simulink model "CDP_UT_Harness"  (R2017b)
settings: Solver=FixedStepDiscrete  StartTime=0.0  StopTime=10.0  FixedStep=0.01  RelTol=1e-3  EnableMultiTasking=on

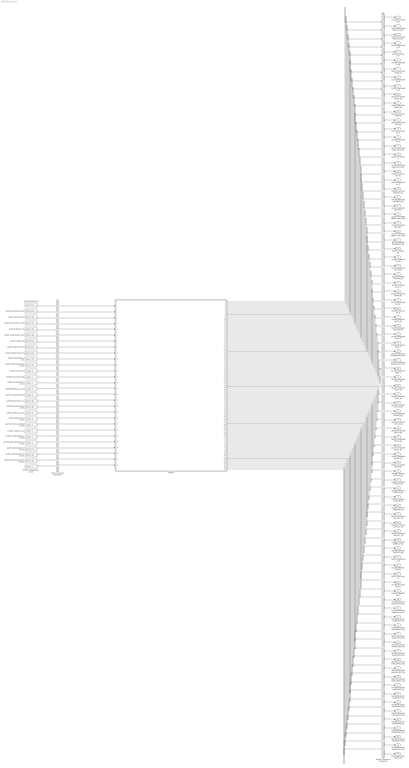
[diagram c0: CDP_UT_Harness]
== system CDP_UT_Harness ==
  CDP_UT : ModelReference  ModelNameDialog=CDP_UT  SimulationMode=Normal  ModelReferenceVersion='M110C20'
  GaISP_AFETempVld_numb : Constant  Value="zeros ( 8  , 1 )"  OutDataTypeStr=uint8  SampleTime=0.01
  GaISP_AFETemp_numb : Constant  Value="zeros ( 8  , 1 )"  OutDataTypeStr=fixdt('ufix16_Sp032_Bn273')  SampleTime=0.01
  GaISP_BusbarTempUpdCnt_numb : Constant  Value="zeros ( 48  , 1 )"  OutDataTypeStr=uint16  SampleTime=0.01
  GaISP_BusbarTempVld_numb : Constant  Value="zeros ( 48  , 1 )"  OutDataTypeStr=uint8  SampleTime=0.01
  GaISP_BusbarTemp_mV : Constant  Value="zeros ( 48  , 1 )"  OutDataTypeStr=uint16  SampleTime=0.01
  GaISP_CMUPCBTempVld_numb : Constant  Value="zeros ( 32  , 1 )"  OutDataTypeStr=uint8  SampleTime=0.01
  GaISP_CMUPCBTemp_mV : Constant  Value="zeros ( 32  , 1 )"  OutDataTypeStr=uint16  SampleTime=0.01
  GaISP_CellBalcOpLine_flg : Constant  Value="zeros ( 112  , 1 )"  OutDataTypeStr=boolean  SampleTime=0.01
  GaISP_CellBalcShrt_flg : Constant  Value="zeros ( 112  , 1 )"  OutDataTypeStr=boolean  SampleTime=0.01
  GaISP_CellBalc_flg : Constant  Value="zeros ( 112  , 1 )"  OutDataTypeStr=boolean  SampleTime=0.01
  GaISP_CellTempUpdCnt_numb : Constant  Value="zeros ( 48  , 1 )"  OutDataTypeStr=uint16  SampleTime=0.01
  GaISP_CellTempVld_numb : Constant  Value="zeros ( 48  , 1 )"  OutDataTypeStr=uint8  SampleTime=0.01
  GaISP_CellTemp_mV : Constant  Value="zeros ( 48  , 1 )"  OutDataTypeStr=uint16  SampleTime=0.01
  GaISP_CellVoltUpdCnt_numb : Constant  Value="zeros ( 112  , 1 )"  OutDataTypeStr=uint16  SampleTime=0.01
  GaISP_CellVoltVld_numb : Constant  Value="zeros ( 112  , 1 )"  OutDataTypeStr=uint8  SampleTime=0.01
  GaISP_CellVolt_mV : Constant  Value="zeros ( 112  , 1 )"  OutDataTypeStr=uint16  SampleTime=0.01
  GaISP_StackVoltVld_numb : Constant  Value="zeros ( 16  , 1 )"  OutDataTypeStr=uint8  SampleTime=0.01
  GaISP_StackVolt_mV : Constant  Value="zeros ( 16  , 1 )"  OutDataTypeStr=uint16  SampleTime=0.01
  GbCTC_ChrgHVMode_flg : Constant  Value="zeros ( 1  , 1 )"  OutDataTypeStr=boolean  SampleTime=0.01
  GbHDP_PackCrntVld_flg : Constant  Value="zeros ( 1  , 1 )"  OutDataTypeStr=boolean  SampleTime=0.01
  GcHDP_PackCrnt_A : Constant  Value="zeros ( 1  , 1 )"  OutDataTypeStr=single  SampleTime=0.01
  GcUDS_BusbarTempNumb_numb : Constant  Value="zeros ( 1  , 1 )"  OutDataTypeStr=uint8  SampleTime=0.01
  GcUDS_CellTempNumb_numb : Constant  Value="zeros ( 1  , 1 )"  OutDataTypeStr=uint8  SampleTime=0.01
  GcUDS_CellVoltNum_numb : Constant  Value="zeros ( 1  , 1 )"  OutDataTypeStr=uint8  SampleTime=0.01
  GeCTC_CtrCtlConnMode_enum : Constant  Value="zeros ( 1  , 1 )"  OutDataTypeStr=uint8  SampleTime=0.01
  GeISP_CmuReIninSts_enum : Constant  Value="zeros ( 1  , 1 )"  OutDataTypeStr=uint8  SampleTime=0.01
  GeMSM_BMUState_enum : Constant  Value="zeros ( 1  , 1 )"  OutDataTypeStr=uint8  SampleTime=0.01
  GeUDS_CapSel_enum : Constant  Value="zeros ( 1  , 1 )"  OutDataTypeStr=uint8  SampleTime=0.01
  Input Conversion Subsystem : Subsystem  Tag=__SLT_ICS__  Description=Signal spec. and routing
  Output Conversion Subsystem : Subsystem  Tag=__SLT_OCS__  Description=Signal spec. and routing
  GcCDP_SumCellVolt_V : Outport  OutDataTypeStr=single  PortDimensions=[1]
  GcCDP_MaxCellVoltNumb_numb : Outport  Port=2  OutDataTypeStr=uint8  PortDimensions=[1]
  GcCDP_MinCellVoltNumb_numb : Outport  Port=3  OutDataTypeStr=uint8  PortDimensions=[1]
  GcCDP_AvgCellVolt_mV : Outport  Port=4  OutDataTypeStr=uint16  PortDimensions=[1]
  GaCDP_CellVolt_mV : Outport  Port=5  OutDataTypeStr=uint16  PortDimensions=[112]
  GaCDP_CellVoltVld_flg : Outport  Port=6  OutDataTypeStr=boolean  PortDimensions=[112]
  GbCDP_SumCellVoltVld_flg : Outport  Port=7  OutDataTypeStr=boolean  PortDimensions=[1]
  GcCDP_MaxCellVolt_mV : Outport  Port=8  OutDataTypeStr=uint16  PortDimensions=[1]
  GcCDP_MinCellVolt_mV : Outport  Port=9  OutDataTypeStr=uint16  PortDimensions=[1]
  GbCDP_CellVoltSelfChck_flg : Outport  Port=10  OutDataTypeStr=boolean  PortDimensions=[1]
  GaCDP_StackVoltHighFlt_flg : Outport  Port=11  OutDataTypeStr=boolean  PortDimensions=[16]
  GaCDP_StackVoltLowFlt_flg : Outport  Port=12  OutDataTypeStr=boolean  PortDimensions=[16]
  GbCDP_AllCellTempVld_flg : Outport  Port=13  OutDataTypeStr=boolean  PortDimensions=[1]
  GcCDP_MaxCellTemp_C : Outport  Port=14  OutDataTypeStr=single  PortDimensions=[1]
  GcCDP_MinCellTemp_C : Outport  Port=15  OutDataTypeStr=single  PortDimensions=[1]
  GcCDP_MaxCellTempNumb_numb : Outport  Port=16  OutDataTypeStr=uint8  PortDimensions=[1]
  GaCDP_CellTemp_C : Outport  Port=17  OutDataTypeStr=single  PortDimensions=[48]
  GcCDP_MinCellTempNumb_numb : Outport  Port=18  OutDataTypeStr=uint8  PortDimensions=[1]
  GaCDP_CellTempVld_flg : Outport  Port=19  OutDataTypeStr=boolean  PortDimensions=[48]
  GcCDP_AvgCellTemp_C : Outport  Port=20  OutDataTypeStr=single  PortDimensions=[1]
  GbCDP_CellTempSelfChck_flg : Outport  Port=21  OutDataTypeStr=boolean  PortDimensions=[1]
  GaCDP_ModuleTempHighFlt_flg : Outport  Port=22  OutDataTypeStr=boolean  PortDimensions=[16]
  GcCDP_MaxCMUPCBTemp_C : Outport  Port=23  OutDataTypeStr=single  PortDimensions=[1]
  GcCDP_MaxCMUPCBTempNumb_numb : Outport  Port=24  OutDataTypeStr=uint8  PortDimensions=[1]
  GcCDP_MinCMUPCBTemp_C : Outport  Port=25  OutDataTypeStr=single  PortDimensions=[1]
  GcCDP_MinCMUPCBTempNumb_numb : Outport  Port=26  OutDataTypeStr=uint8  PortDimensions=[1]
  GbCDP_CMUPCBTempHighFlt_flg : Outport  Port=27  OutDataTypeStr=boolean  PortDimensions=[1]
  GaCDP_CellBalc_flg : Outport  Port=28  OutDataTypeStr=boolean  PortDimensions=[112]
  GaCDP_CellBalcShrt_flg : Outport  Port=29  OutDataTypeStr=boolean  PortDimensions=[112]
  GaCDP_CellBalcOpLine_flg : Outport  Port=30  OutDataTypeStr=boolean  PortDimensions=[112]
  GaCDP_CMUPCBTempVld_flg : Outport  Port=31  OutDataTypeStr=boolean  PortDimensions=[32]
  GaCDP_CMUPCBTemp_C : Outport  Port=32  OutDataTypeStr=single  PortDimensions=[32]
  GbCDP_SumModelVoltVld_flg : Outport  Port=33  OutDataTypeStr=boolean  PortDimensions=[1]
  GcCDP_SumModelVolt_V : Outport  Port=34  OutDataTypeStr=single  PortDimensions=[1]
  GaCDP_BusbarTemp_C : Outport  Port=35  OutDataTypeStr=single  PortDimensions=[48]
  GaCDP_BusbarTempVld_flg : Outport  Port=36  OutDataTypeStr=boolean  PortDimensions=[48]
  GbCDP_AllBusbarTempVld_flg : Outport  Port=37  OutDataTypeStr=boolean  PortDimensions=[1]
  GcCDP_MaxBusbarTemp_C : Outport  Port=38  OutDataTypeStr=single  PortDimensions=[1]
  GcCDP_MinBusbarTemp_C : Outport  Port=39  OutDataTypeStr=single  PortDimensions=[1]
  GcCDP_MaxBusbarTempNumb_numb : Outport  Port=40  OutDataTypeStr=uint8  PortDimensions=[1]
  GcCDP_MinBusbarTempNumb_numb : Outport  Port=41  OutDataTypeStr=uint8  PortDimensions=[1]
  GcCDP_AvgBusbarTemp_C : Outport  Port=42  OutDataTypeStr=single  PortDimensions=[1]
  GbCDP_CellVoltHiFltLv3_flg : Outport  Port=43  OutDataTypeStr=boolean  PortDimensions=[1]
  GbCDP_CellVoltHiFltLv2_flg : Outport  Port=44  OutDataTypeStr=boolean  PortDimensions=[1]
  GbCDP_CellVoltHiFltLv1_flg : Outport  Port=45  OutDataTypeStr=boolean  PortDimensions=[1]
  GbCDP_CellVoltLowFltLv3_flg : Outport  Port=46  OutDataTypeStr=boolean  PortDimensions=[1]
  GbCDP_CellVoltLowFltLv2_flg : Outport  Port=47  OutDataTypeStr=boolean  PortDimensions=[1]
  GbCDP_CellVoltLowFltLv1_flg : Outport  Port=48  OutDataTypeStr=boolean  PortDimensions=[1]
  GbCDP_CellVoltDiffFltLv3_flg : Outport  Port=49  OutDataTypeStr=boolean  PortDimensions=[1]
  GbCDP_CellVoltDiffFltLv2_flg : Outport  Port=50  OutDataTypeStr=boolean  PortDimensions=[1]
  GbCDP_CellVoltDiffFltLv1_flg : Outport  Port=51  OutDataTypeStr=boolean  PortDimensions=[1]
  GbCDP_CellVoltRngLowFlt_flg : Outport  Port=52  OutDataTypeStr=boolean  PortDimensions=[1]
  GbCDP_CellVoltRngHiFlt_flg : Outport  Port=53  OutDataTypeStr=boolean  PortDimensions=[1]
  GbCDP_CellTempHiFltLv3_flg : Outport  Port=54  OutDataTypeStr=boolean  PortDimensions=[1]
  GbCDP_CellTempHiFltLv2_flg : Outport  Port=55  OutDataTypeStr=boolean  PortDimensions=[1]
  GbCDP_CellTempHiFltLv1_flg : Outport  Port=56  OutDataTypeStr=boolean  PortDimensions=[1]
  GbCDP_CellTempRngHiFlt_flg : Outport  Port=57  OutDataTypeStr=boolean  PortDimensions=[1]
  GbCDP_CellTempRngLowFlt_flg : Outport  Port=58  OutDataTypeStr=boolean  PortDimensions=[1]
  GbCDP_CellTempLowFltLv3_flg : Outport  Port=59  OutDataTypeStr=boolean  PortDimensions=[1]
  GbCDP_CellTempLowFltLv2_flg : Outport  Port=60  OutDataTypeStr=boolean  PortDimensions=[1]
  GbCDP_CellTempLowFltLv1_flg : Outport  Port=61  OutDataTypeStr=boolean  PortDimensions=[1]
  GbCDP_CellTempDiffFltLv2_flg : Outport  Port=62  OutDataTypeStr=boolean  PortDimensions=[1]
  GbCDP_CellTempDiffFltLv1_flg : Outport  Port=63  OutDataTypeStr=boolean  PortDimensions=[1]
  GaCDP_ModuleVolt_mV : Outport  Port=64  OutDataTypeStr=uint16  PortDimensions=[16]
  GaCDP_AFETempVld_flg : Outport  Port=65  OutDataTypeStr=boolean  PortDimensions=[8]
  GaCDP_AFETemp_C : Outport  Port=66  OutDataTypeStr=single  PortDimensions=[8]
  GcCDP_MaxAFETemp_C : Outport  Port=67  OutDataTypeStr=single  PortDimensions=[1]
  GcCDP_MinAFETemp_C : Outport  Port=68  OutDataTypeStr=single  PortDimensions=[1]
  GcCDP_MaxAFETempNumb_numb : Outport  Port=69  OutDataTypeStr=uint8  PortDimensions=[1]
  GcCDP_MinAFETempNumb_numb : Outport  Port=70  OutDataTypeStr=uint8  PortDimensions=[1]
  GbCDP_BusbarTempHiFltLv3_flg : Outport  Port=71  OutDataTypeStr=boolean  PortDimensions=[1]
  GbCDP_BusbarTempLowFltLv3_flg : Outport  Port=72  OutDataTypeStr=boolean  PortDimensions=[1]
  GbCDP_ChrgCellTempHiFltLv3_flg : Outport  Port=73  OutDataTypeStr=boolean  PortDimensions=[1]
  GbCDP_ChrgCellTempHiFltLv2_flg : Outport  Port=74  OutDataTypeStr=boolean  PortDimensions=[1]
  GbCDP_ChrgCellTempHiFltLv1_flg : Outport  Port=75  OutDataTypeStr=boolean  PortDimensions=[1]
  GbCDP_ChrgCellTempLowFltLv3_flg : Outport  Port=76  OutDataTypeStr=boolean  PortDimensions=[1]
  GbCDP_ChrgCellTempLowFltLv2_flg : Outport  Port=77  OutDataTypeStr=boolean  PortDimensions=[1]
  GbCDP_ChrgCellTempLowFltLv1_flg : Outport  Port=78  OutDataTypeStr=boolean  PortDimensions=[1]
  GbCDP_BusbarTempHiFltLv2_flg : Outport  Port=79  OutDataTypeStr=boolean  PortDimensions=[1]
  GbCDP_BusbarTempHiFltLv1_flg : Outport  Port=80  OutDataTypeStr=boolean  PortDimensions=[1]
  GbCDP_BusbarTempLowFltLv2_flg : Outport  Port=81  OutDataTypeStr=boolean  PortDimensions=[1]
  GbCDP_BusbarTempLowFltLv1_flg : Outport  Port=82  OutDataTypeStr=boolean  PortDimensions=[1]
  GbCDP_BusbarTempRngHiFlt_flg : Outport  Port=83  OutDataTypeStr=boolean  PortDimensions=[1]
  GbCDP_BusbarTempRngLowFlt_flg : Outport  Port=84  OutDataTypeStr=boolean  PortDimensions=[1]
  GbCDP_BusbarTempDiffFltLv2_flg : Outport  Port=85  OutDataTypeStr=boolean  PortDimensions=[1]
  GbCDP_BusbarTempDiffFltLv1_flg : Outport  Port=86  OutDataTypeStr=boolean  PortDimensions=[1]
  GbCDP_AFETempHighFlt_flg : Outport  Port=87  OutDataTypeStr=boolean  PortDimensions=[1]
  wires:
  GaISP_CellVolt_mV/1 -> Input Conversion Subsystem/1(Inport_1)
  GaISP_CellVoltVld_numb/1 -> Input Conversion Subsystem/2(Inport_2)
  GaISP_StackVolt_mV/1 -> Input Conversion Subsystem/3(Inport_3)
  GaISP_StackVoltVld_numb/1 -> Input Conversion Subsystem/4(Inport_4)
  GaISP_CellTemp_mV/1 -> Input Conversion Subsystem/5(Inport_5)
  GaISP_CellTempVld_numb/1 -> Input Conversion Subsystem/6(Inport_6)
  GaISP_CellBalc_flg/1 -> Input Conversion Subsystem/7(Inport_7)
  GaISP_CellBalcShrt_flg/1 -> Input Conversion Subsystem/8(Inport_8)
  GaISP_CellBalcOpLine_flg/1 -> Input Conversion Subsystem/9(Inport_9)
  GaISP_CMUPCBTemp_mV/1 -> Input Conversion Subsystem/10(Inport_10)
  GaISP_CMUPCBTempVld_numb/1 -> Input Conversion Subsystem/11(Inport_11)
  GcHDP_PackCrnt_A/1 -> Input Conversion Subsystem/12(Inport_12)
  GbHDP_PackCrntVld_flg/1 -> Input Conversion Subsystem/13(Inport_13)
  GeISP_CmuReIninSts_enum/1 -> Input Conversion Subsystem/14(Inport_14)
  GeMSM_BMUState_enum/1 -> Input Conversion Subsystem/15(Inport_15)
  GbCTC_ChrgHVMode_flg/1 -> Input Conversion Subsystem/16(Inport_16)
  GaISP_BusbarTemp_mV/1 -> Input Conversion Subsystem/17(Inport_17)
  GaISP_BusbarTempVld_numb/1 -> Input Conversion Subsystem/18(Inport_18)
  GaISP_AFETemp_numb/1 -> Input Conversion Subsystem/19(Inport_19)
  GaISP_AFETempVld_numb/1 -> Input Conversion Subsystem/20(Inport_20)
  GeCTC_CtrCtlConnMode_enum/1 -> Input Conversion Subsystem/21(Inport_21)
  GeUDS_CapSel_enum/1 -> Input Conversion Subsystem/22(Inport_22)
  GcUDS_CellTempNumb_numb/1 -> Input Conversion Subsystem/23(Inport_23)
  GcUDS_BusbarTempNumb_numb/1 -> Input Conversion Subsystem/24(Inport_24)
  GaISP_CellVoltUpdCnt_numb/1 -> Input Conversion Subsystem/25(Inport_25)
  GaISP_CellTempUpdCnt_numb/1 -> Input Conversion Subsystem/26(Inport_26)
  GaISP_BusbarTempUpdCnt_numb/1 -> Input Conversion Subsystem/27(Inport_27)
  GcUDS_CellVoltNum_numb/1 -> Input Conversion Subsystem/28(Inport_28)
  Output Conversion Subsystem/1(Outport_1) -> GcCDP_SumCellVolt_V/1
  Output Conversion Subsystem/2(Outport_2) -> GcCDP_MaxCellVoltNumb_numb/1
  Output Conversion Subsystem/3(Outport_3) -> GcCDP_MinCellVoltNumb_numb/1
  Output Conversion Subsystem/4(Outport_4) -> GcCDP_AvgCellVolt_mV/1
  Output Conversion Subsystem/5(Outport_5) -> GaCDP_CellVolt_mV/1
  Output Conversion Subsystem/6(Outport_6) -> GaCDP_CellVoltVld_flg/1
  Output Conversion Subsystem/7(Outport_7) -> GbCDP_SumCellVoltVld_flg/1
  Output Conversion Subsystem/8(Outport_8) -> GcCDP_MaxCellVolt_mV/1
  Output Conversion Subsystem/9(Outport_9) -> GcCDP_MinCellVolt_mV/1
  Output Conversion Subsystem/10(Outport_10) -> GbCDP_CellVoltSelfChck_flg/1
  Output Conversion Subsystem/11(Outport_11) -> GaCDP_StackVoltHighFlt_flg/1
  Output Conversion Subsystem/12(Outport_12) -> GaCDP_StackVoltLowFlt_flg/1
  Output Conversion Subsystem/13(Outport_13) -> GbCDP_AllCellTempVld_flg/1
  Output Conversion Subsystem/14(Outport_14) -> GcCDP_MaxCellTemp_C/1
  Output Conversion Subsystem/15(Outport_15) -> GcCDP_MinCellTemp_C/1
  Output Conversion Subsystem/16(Outport_16) -> GcCDP_MaxCellTempNumb_numb/1
  Output Conversion Subsystem/17(Outport_17) -> GaCDP_CellTemp_C/1
  Output Conversion Subsystem/18(Outport_18) -> GcCDP_MinCellTempNumb_numb/1
  Output Conversion Subsystem/19(Outport_19) -> GaCDP_CellTempVld_flg/1
  Output Conversion Subsystem/20(Outport_20) -> GcCDP_AvgCellTemp_C/1
  Output Conversion Subsystem/21(Outport_21) -> GbCDP_CellTempSelfChck_flg/1
  Output Conversion Subsystem/22(Outport_22) -> GaCDP_ModuleTempHighFlt_flg/1
  Output Conversion Subsystem/23(Outport_23) -> GcCDP_MaxCMUPCBTemp_C/1
  Output Conversion Subsystem/24(Outport_24) -> GcCDP_MaxCMUPCBTempNumb_numb/1
  Output Conversion Subsystem/25(Outport_25) -> GcCDP_MinCMUPCBTemp_C/1
  Output Conversion Subsystem/26(Outport_26) -> GcCDP_MinCMUPCBTempNumb_numb/1
  Output Conversion Subsystem/27(Outport_27) -> GbCDP_CMUPCBTempHighFlt_flg/1
  Output Conversion Subsystem/28(Outport_28) -> GaCDP_CellBalc_flg/1
  Output Conversion Subsystem/29(Outport_29) -> GaCDP_CellBalcShrt_flg/1
  Output Conversion Subsystem/30(Outport_30) -> GaCDP_CellBalcOpLine_flg/1
  Output Conversion Subsystem/31(Outport_31) -> GaCDP_CMUPCBTempVld_flg/1
  Output Conversion Subsystem/32(Outport_32) -> GaCDP_CMUPCBTemp_C/1
  Output Conversion Subsystem/33(Outport_33) -> GbCDP_SumModelVoltVld_flg/1
  Output Conversion Subsystem/34(Outport_34) -> GcCDP_SumModelVolt_V/1
  Output Conversion Subsystem/35(Outport_35) -> GaCDP_BusbarTemp_C/1
  Output Conversion Subsystem/36(Outport_36) -> GaCDP_BusbarTempVld_flg/1
  Output Conversion Subsystem/37(Outport_37) -> GbCDP_AllBusbarTempVld_flg/1
  Output Conversion Subsystem/38(Outport_38) -> GcCDP_MaxBusbarTemp_C/1
  Output Conversion Subsystem/39(Outport_39) -> GcCDP_MinBusbarTemp_C/1
  Output Conversion Subsystem/40(Outport_40) -> GcCDP_MaxBusbarTempNumb_numb/1
  Output Conversion Subsystem/41(Outport_41) -> GcCDP_MinBusbarTempNumb_numb/1
  Output Conversion Subsystem/42(Outport_42) -> GcCDP_AvgBusbarTemp_C/1
  Output Conversion Subsystem/43(Outport_43) -> GbCDP_CellVoltHiFltLv3_flg/1
  Output Conversion Subsystem/44(Outport_44) -> GbCDP_CellVoltHiFltLv2_flg/1
  Output Conversion Subsystem/45(Outport_45) -> GbCDP_CellVoltHiFltLv1_flg/1
  Output Conversion Subsystem/46(Outport_46) -> GbCDP_CellVoltLowFltLv3_flg/1
  Output Conversion Subsystem/47(Outport_47) -> GbCDP_CellVoltLowFltLv2_flg/1
  Output Conversion Subsystem/48(Outport_48) -> GbCDP_CellVoltLowFltLv1_flg/1
  Output Conversion Subsystem/49(Outport_49) -> GbCDP_CellVoltDiffFltLv3_flg/1
  Output Conversion Subsystem/50(Outport_50) -> GbCDP_CellVoltDiffFltLv2_flg/1
  Output Conversion Subsystem/51(Outport_51) -> GbCDP_CellVoltDiffFltLv1_flg/1
  Output Conversion Subsystem/52(Outport_52) -> GbCDP_CellVoltRngLowFlt_flg/1
  Output Conversion Subsystem/53(Outport_53) -> GbCDP_CellVoltRngHiFlt_flg/1
  Output Conversion Subsystem/54(Outport_54) -> GbCDP_CellTempHiFltLv3_flg/1
  Output Conversion Subsystem/55(Outport_55) -> GbCDP_CellTempHiFltLv2_flg/1
  Output Conversion Subsystem/56(Outport_56) -> GbCDP_CellTempHiFltLv1_flg/1
  Output Conversion Subsystem/57(Outport_57) -> GbCDP_CellTempRngHiFlt_flg/1
  Output Conversion Subsystem/58(Outport_58) -> GbCDP_CellTempRngLowFlt_flg/1
  Output Conversion Subsystem/59(Outport_59) -> GbCDP_CellTempLowFltLv3_flg/1
  Output Conversion Subsystem/60(Outport_60) -> GbCDP_CellTempLowFltLv2_flg/1
  Output Conversion Subsystem/61(Outport_61) -> GbCDP_CellTempLowFltLv1_flg/1
  Output Conversion Subsystem/62(Outport_62) -> GbCDP_CellTempDiffFltLv2_flg/1
  Output Conversion Subsystem/63(Outport_63) -> GbCDP_CellTempDiffFltLv1_flg/1
  Output Conversion Subsystem/64(Outport_64) -> GaCDP_ModuleVolt_mV/1
  Output Conversion Subsystem/65(Outport_65) -> GaCDP_AFETempVld_flg/1
  Output Conversion Subsystem/66(Outport_66) -> GaCDP_AFETemp_C/1
  Output Conversion Subsystem/67(Outport_67) -> GcCDP_MaxAFETemp_C/1
  Output Conversion Subsystem/68(Outport_68) -> GcCDP_MinAFETemp_C/1
  Output Conversion Subsystem/69(Outport_69) -> GcCDP_MaxAFETempNumb_numb/1
  Output Conversion Subsystem/70(Outport_70) -> GcCDP_MinAFETempNumb_numb/1
  Output Conversion Subsystem/71(Outport_71) -> GbCDP_BusbarTempHiFltLv3_flg/1
  Output Conversion Subsystem/72(Outport_72) -> GbCDP_BusbarTempLowFltLv3_flg/1
  Output Conversion Subsystem/73(Outport_73) -> GbCDP_ChrgCellTempHiFltLv3_flg/1
  Output Conversion Subsystem/74(Outport_74) -> GbCDP_ChrgCellTempHiFltLv2_flg/1
  Output Conversion Subsystem/75(Outport_75) -> GbCDP_ChrgCellTempHiFltLv1_flg/1
  Output Conversion Subsystem/76(Outport_76) -> GbCDP_ChrgCellTempLowFltLv3_flg/1
  Output Conversion Subsystem/77(Outport_77) -> GbCDP_ChrgCellTempLowFltLv2_flg/1
  Output Conversion Subsystem/78(Outport_78) -> GbCDP_ChrgCellTempLowFltLv1_flg/1
  Output Conversion Subsystem/79(Outport_79) -> GbCDP_BusbarTempHiFltLv2_flg/1
  Output Conversion Subsystem/80(Outport_80) -> GbCDP_BusbarTempHiFltLv1_flg/1
  Output Conversion Subsystem/81(Outport_81) -> GbCDP_BusbarTempLowFltLv2_flg/1
  Output Conversion Subsystem/82(Outport_82) -> GbCDP_BusbarTempLowFltLv1_flg/1
  Output Conversion Subsystem/83(Outport_83) -> GbCDP_BusbarTempRngHiFlt_flg/1
  Output Conversion Subsystem/84(Outport_84) -> GbCDP_BusbarTempRngLowFlt_flg/1
  Output Conversion Subsystem/85(Outport_85) -> GbCDP_BusbarTempDiffFltLv2_flg/1
  Output Conversion Subsystem/86(Outport_86) -> GbCDP_BusbarTempDiffFltLv1_flg/1
  Output Conversion Subsystem/87(Outport_87) -> GbCDP_AFETempHighFlt_flg/1
  Input Conversion Subsystem/1(Outport_1) -> CDP_UT/1
  Input Conversion Subsystem/2(Outport_2) -> CDP_UT/2
  Input Conversion Subsystem/3(Outport_3) -> CDP_UT/3
  Input Conversion Subsystem/4(Outport_4) -> CDP_UT/4
  Input Conversion Subsystem/5(Outport_5) -> CDP_UT/5
  Input Conversion Subsystem/6(Outport_6) -> CDP_UT/6
  Input Conversion Subsystem/7(Outport_7) -> CDP_UT/7
  Input Conversion Subsystem/8(Outport_8) -> CDP_UT/8
  Input Conversion Subsystem/9(Outport_9) -> CDP_UT/9
  Input Conversion Subsystem/10(Outport_10) -> CDP_UT/10
  Input Conversion Subsystem/11(Outport_11) -> CDP_UT/11
  Input Conversion Subsystem/12(Outport_12) -> CDP_UT/12
  Input Conversion Subsystem/13(Outport_13) -> CDP_UT/13
  Input Conversion Subsystem/14(Outport_14) -> CDP_UT/14
  Input Conversion Subsystem/15(Outport_15) -> CDP_UT/15
  Input Conversion Subsystem/16(Outport_16) -> CDP_UT/16
  Input Conversion Subsystem/17(Outport_17) -> CDP_UT/17
  Input Conversion Subsystem/18(Outport_18) -> CDP_UT/18
  Input Conversion Subsystem/19(Outport_19) -> CDP_UT/19
  Input Conversion Subsystem/20(Outport_20) -> CDP_UT/20
  Input Conversion Subsystem/21(Outport_21) -> CDP_UT/21
  Input Conversion Subsystem/22(Outport_22) -> CDP_UT/22
  Input Conversion Subsystem/23(Outport_23) -> CDP_UT/23
  Input Conversion Subsystem/24(Outport_24) -> CDP_UT/24
  Input Conversion Subsystem/25(Outport_25) -> CDP_UT/25
  Input Conversion Subsystem/26(Outport_26) -> CDP_UT/26
  Input Conversion Subsystem/27(Outport_27) -> CDP_UT/27
  Input Conversion Subsystem/28(Outport_28) -> CDP_UT/28
  CDP_UT/1 -> Output Conversion Subsystem/1(Inport_1)
  CDP_UT/2 -> Output Conversion Subsystem/2(Inport_2)
  CDP_UT/3 -> Output Conversion Subsystem/3(Inport_3)
  CDP_UT/4 -> Output Conversion Subsystem/4(Inport_4)
  CDP_UT/5 -> Output Conversion Subsystem/5(Inport_5)
  CDP_UT/6 -> Output Conversion Subsystem/6(Inport_6)
  CDP_UT/7 -> Output Conversion Subsystem/7(Inport_7)
  CDP_UT/8 -> Output Conversion Subsystem/8(Inport_8)
  CDP_UT/9 -> Output Conversion Subsystem/9(Inport_9)
  CDP_UT/10 -> Output Conversion Subsystem/10(Inport_10)
  CDP_UT/11 -> Output Conversion Subsystem/11(Inport_11)
  CDP_UT/12 -> Output Conversion Subsystem/12(Inport_12)
  CDP_UT/13 -> Output Conversion Subsystem/13(Inport_13)
  CDP_UT/14 -> Output Conversion Subsystem/14(Inport_14)
  CDP_UT/15 -> Output Conversion Subsystem/15(Inport_15)
  CDP_UT/16 -> Output Conversion Subsystem/16(Inport_16)
  CDP_UT/17 -> Output Conversion Subsystem/17(Inport_17)
  CDP_UT/18 -> Output Conversion Subsystem/18(Inport_18)
  CDP_UT/19 -> Output Conversion Subsystem/19(Inport_19)
  CDP_UT/20 -> Output Conversion Subsystem/20(Inport_20)
  CDP_UT/21 -> Output Conversion Subsystem/21(Inport_21)
  CDP_UT/22 -> Output Conversion Subsystem/22(Inport_22)
  CDP_UT/23 -> Output Conversion Subsystem/23(Inport_23)
  CDP_UT/24 -> Output Conversion Subsystem/24(Inport_24)
  CDP_UT/25 -> Output Conversion Subsystem/25(Inport_25)
  CDP_UT/26 -> Output Conversion Subsystem/26(Inport_26)
  CDP_UT/27 -> Output Conversion Subsystem/27(Inport_27)
  CDP_UT/28 -> Output Conversion Subsystem/28(Inport_28)
  CDP_UT/29 -> Output Conversion Subsystem/29(Inport_29)
  CDP_UT/30 -> Output Conversion Subsystem/30(Inport_30)
  CDP_UT/31 -> Output Conversion Subsystem/31(Inport_31)
  CDP_UT/32 -> Output Conversion Subsystem/32(Inport_32)
  CDP_UT/33 -> Output Conversion Subsystem/33(Inport_33)
  CDP_UT/34 -> Output Conversion Subsystem/34(Inport_34)
  CDP_UT/35 -> Output Conversion Subsystem/35(Inport_35)
  CDP_UT/36 -> Output Conversion Subsystem/36(Inport_36)
  CDP_UT/37 -> Output Conversion Subsystem/37(Inport_37)
  CDP_UT/38 -> Output Conversion Subsystem/38(Inport_38)
  CDP_UT/39 -> Output Conversion Subsystem/39(Inport_39)
  CDP_UT/40 -> Output Conversion Subsystem/40(Inport_40)
  CDP_UT/41 -> Output Conversion Subsystem/41(Inport_41)
  CDP_UT/42 -> Output Conversion Subsystem/42(Inport_42)
  CDP_UT/43 -> Output Conversion Subsystem/43(Inport_43)
  CDP_UT/44 -> Output Conversion Subsystem/44(Inport_44)
  CDP_UT/45 -> Output Conversion Subsystem/45(Inport_45)
  CDP_UT/46 -> Output Conversion Subsystem/46(Inport_46)
  CDP_UT/47 -> Output Conversion Subsystem/47(Inport_47)
  CDP_UT/48 -> Output Conversion Subsystem/48(Inport_48)
  CDP_UT/49 -> Output Conversion Subsystem/49(Inport_49)
  CDP_UT/50 -> Output Conversion Subsystem/50(Inport_50)
  CDP_UT/51 -> Output Conversion Subsystem/51(Inport_51)
  CDP_UT/52 -> Output Conversion Subsystem/52(Inport_52)
  CDP_UT/53 -> Output Conversion Subsystem/53(Inport_53)
  CDP_UT/54 -> Output Conversion Subsystem/54(Inport_54)
  CDP_UT/55 -> Output Conversion Subsystem/55(Inport_55)
  CDP_UT/56 -> Output Conversion Subsystem/56(Inport_56)
  CDP_UT/57 -> Output Conversion Subsystem/57(Inport_57)
  CDP_UT/58 -> Output Conversion Subsystem/58(Inport_58)
  CDP_UT/59 -> Output Conversion Subsystem/59(Inport_59)
  CDP_UT/60 -> Output Conversion Subsystem/60(Inport_60)
  CDP_UT/61 -> Output Conversion Subsystem/61(Inport_61)
  CDP_UT/62 -> Output Conversion Subsystem/62(Inport_62)
  CDP_UT/63 -> Output Conversion Subsystem/63(Inport_63)
  CDP_UT/64 -> Output Conversion Subsystem/64(Inport_64)
  CDP_UT/65 -> Output Conversion Subsystem/65(Inport_65)
  CDP_UT/66 -> Output Conversion Subsystem/66(Inport_66)
  CDP_UT/67 -> Output Conversion Subsystem/67(Inport_67)
  CDP_UT/68 -> Output Conversion Subsystem/68(Inport_68)
  CDP_UT/69 -> Output Conversion Subsystem/69(Inport_69)
  CDP_UT/70 -> Output Conversion Subsystem/70(Inport_70)
  CDP_UT/71 -> Output Conversion Subsystem/71(Inport_71)
  CDP_UT/72 -> Output Conversion Subsystem/72(Inport_72)
  CDP_UT/73 -> Output Conversion Subsystem/73(Inport_73)
  CDP_UT/74 -> Output Conversion Subsystem/74(Inport_74)
  CDP_UT/75 -> Output Conversion Subsystem/75(Inport_75)
  CDP_UT/76 -> Output Conversion Subsystem/76(Inport_76)
  CDP_UT/77 -> Output Conversion Subsystem/77(Inport_77)
  CDP_UT/78 -> Output Conversion Subsystem/78(Inport_78)
  CDP_UT/79 -> Output Conversion Subsystem/79(Inport_79)
  CDP_UT/80 -> Output Conversion Subsystem/80(Inport_80)
  CDP_UT/81 -> Output Conversion Subsystem/81(Inport_81)
  CDP_UT/82 -> Output Conversion Subsystem/82(Inport_82)
  CDP_UT/83 -> Output Conversion Subsystem/83(Inport_83)
  CDP_UT/84 -> Output Conversion Subsystem/84(Inport_84)
  CDP_UT/85 -> Output Conversion Subsystem/85(Inport_85)
  CDP_UT/86 -> Output Conversion Subsystem/86(Inport_86)
  CDP_UT/87 -> Output Conversion Subsystem/87(Inport_87)

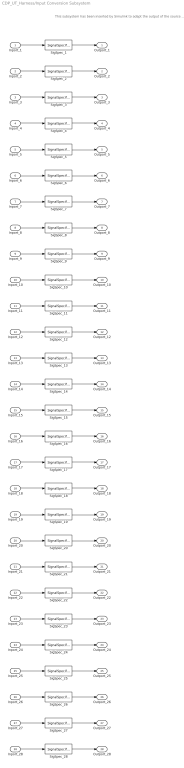
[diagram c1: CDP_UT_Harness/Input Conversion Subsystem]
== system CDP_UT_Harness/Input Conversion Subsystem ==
  note: This subsystem has been inserted by Simulink to adapt the output of the source blocks to the interface required by the harnessed component. Modifying the contents of this subsystem may result in compilation and simulation failure.
  Inport_1 : Inport
  Inport_2 : Inport  Port=2
  Inport_3 : Inport  Port=3
  Inport_4 : Inport  Port=4
  Inport_5 : Inport  Port=5
  Inport_6 : Inport  Port=6
  Inport_7 : Inport  Port=7
  Inport_8 : Inport  Port=8
  Inport_9 : Inport  Port=9
  Inport_10 : Inport  Port=10
  Inport_11 : Inport  Port=11
  Inport_12 : Inport  Port=12
  Inport_13 : Inport  Port=13
  Inport_14 : Inport  Port=14
  Inport_15 : Inport  Port=15
  Inport_16 : Inport  Port=16
  Inport_17 : Inport  Port=17
  Inport_18 : Inport  Port=18
  Inport_19 : Inport  Port=19
  Inport_20 : Inport  Port=20
  Inport_21 : Inport  Port=21
  Inport_22 : Inport  Port=22
  Inport_23 : Inport  Port=23
  Inport_24 : Inport  Port=24
  Inport_25 : Inport  Port=25
  Inport_26 : Inport  Port=26
  Inport_27 : Inport  Port=27
  Inport_28 : Inport  Port=28
  SigSpec_1 : SignalSpecification  OutDataTypeStr=uint16  Unit=mV  Dimensions=[112]  SampleTime=0.01
  SigSpec_10 : SignalSpecification  OutDataTypeStr=uint16  Unit=mV  Dimensions=[32]  SampleTime=0.01
  SigSpec_11 : SignalSpecification  OutDataTypeStr=uint8  Unit=numb  Dimensions=[32]  SampleTime=0.01
  SigSpec_12 : SignalSpecification  OutDataTypeStr=single  Unit=A  Dimensions=[1]  SampleTime=0.01
  SigSpec_13 : SignalSpecification  OutDataTypeStr=boolean  Unit=flag  Dimensions=[1]  SampleTime=0.01
  SigSpec_{14..15,21..22} (4 alike) : SignalSpecification  OutDataTypeStr=uint8  Unit=enum  Dimensions=[1]  SampleTime=0.01
  SigSpec_16 : SignalSpecification  OutDataTypeStr=boolean  Unit=flag  Dimensions=[1]  SampleTime=0.01
  SigSpec_17 : SignalSpecification  OutDataTypeStr=uint16  Unit=mV  Dimensions=[48]  SampleTime=0.01
  SigSpec_18 : SignalSpecification  OutDataTypeStr=uint8  Unit=numb  Dimensions=[48]  SampleTime=0.01
  SigSpec_19 : SignalSpecification  OutDataTypeStr=fixdt('ufix16_Sp032_Bn273')  Unit=numb  Dimensions=[8]  SampleTime=0.01
  SigSpec_2 : SignalSpecification  OutDataTypeStr=uint8  Unit=numb  Dimensions=[112]  SampleTime=0.01
  SigSpec_20 : SignalSpecification  OutDataTypeStr=uint8  Unit=numb  Dimensions=[8]  SampleTime=0.01
  SigSpec_23 : SignalSpecification  OutDataTypeStr=uint8  Unit=numb  Dimensions=[1]  SampleTime=0.01
  SigSpec_24 : SignalSpecification  OutDataTypeStr=uint8  Unit=numb  Dimensions=[1]  SampleTime=0.01
  SigSpec_25 : SignalSpecification  OutDataTypeStr=uint16  Unit=numb  Dimensions=[112]  SampleTime=0.01
  SigSpec_26 : SignalSpecification  OutDataTypeStr=uint16  Unit=numb  Dimensions=[48]  SampleTime=0.01
  SigSpec_27 : SignalSpecification  OutDataTypeStr=uint16  Unit=numb  Dimensions=[48]  SampleTime=0.01
  SigSpec_28 : SignalSpecification  OutDataTypeStr=uint8  Unit=numb  Dimensions=[1]  SampleTime=0.01
  SigSpec_3 : SignalSpecification  OutDataTypeStr=uint16  Unit=mV  Dimensions=[16]  SampleTime=0.01
  SigSpec_4 : SignalSpecification  OutDataTypeStr=uint8  Unit=numb  Dimensions=[16]  SampleTime=0.01
  SigSpec_5 : SignalSpecification  OutDataTypeStr=uint16  Unit=mV  Dimensions=[48]  SampleTime=0.01
  SigSpec_6 : SignalSpecification  OutDataTypeStr=uint8  Unit=numb  Dimensions=[48]  SampleTime=0.01
  SigSpec_7 : SignalSpecification  OutDataTypeStr=boolean  Unit=flag  Dimensions=[112]  SampleTime=0.01
  SigSpec_8 : SignalSpecification  OutDataTypeStr=boolean  Unit=flag  Dimensions=[112]  SampleTime=0.01
  SigSpec_9 : SignalSpecification  OutDataTypeStr=boolean  Unit=flag  Dimensions=[112]  SampleTime=0.01
  Outport_1 : Outport
  Outport_2 : Outport  Port=2
  Outport_3 : Outport  Port=3
  Outport_4 : Outport  Port=4
  Outport_5 : Outport  Port=5
  Outport_6 : Outport  Port=6
  Outport_7 : Outport  Port=7
  Outport_8 : Outport  Port=8
  Outport_9 : Outport  Port=9
  Outport_10 : Outport  Port=10
  Outport_11 : Outport  Port=11
  Outport_12 : Outport  Port=12
  Outport_13 : Outport  Port=13
  Outport_14 : Outport  Port=14
  Outport_15 : Outport  Port=15
  Outport_16 : Outport  Port=16
  Outport_17 : Outport  Port=17
  Outport_18 : Outport  Port=18
  Outport_19 : Outport  Port=19
  Outport_20 : Outport  Port=20
  Outport_21 : Outport  Port=21
  Outport_22 : Outport  Port=22
  Outport_23 : Outport  Port=23
  Outport_24 : Outport  Port=24
  Outport_25 : Outport  Port=25
  Outport_26 : Outport  Port=26
  Outport_27 : Outport  Port=27
  Outport_28 : Outport  Port=28
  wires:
  SigSpec_1/1 -> Outport_1/1
  Inport_1/1 -> SigSpec_1/1
  SigSpec_2/1 -> Outport_2/1
  Inport_2/1 -> SigSpec_2/1
  SigSpec_3/1 -> Outport_3/1
  Inport_3/1 -> SigSpec_3/1
  SigSpec_4/1 -> Outport_4/1
  Inport_4/1 -> SigSpec_4/1
  SigSpec_5/1 -> Outport_5/1
  Inport_5/1 -> SigSpec_5/1
  SigSpec_6/1 -> Outport_6/1
  Inport_6/1 -> SigSpec_6/1
  SigSpec_7/1 -> Outport_7/1
  Inport_7/1 -> SigSpec_7/1
  SigSpec_8/1 -> Outport_8/1
  Inport_8/1 -> SigSpec_8/1
  SigSpec_9/1 -> Outport_9/1
  Inport_9/1 -> SigSpec_9/1
  SigSpec_10/1 -> Outport_10/1
  Inport_10/1 -> SigSpec_10/1
  SigSpec_11/1 -> Outport_11/1
  Inport_11/1 -> SigSpec_11/1
  SigSpec_12/1 -> Outport_12/1
  Inport_12/1 -> SigSpec_12/1
  SigSpec_13/1 -> Outport_13/1
  Inport_13/1 -> SigSpec_13/1
  SigSpec_14/1 -> Outport_14/1
  Inport_14/1 -> SigSpec_14/1
  SigSpec_15/1 -> Outport_15/1
  Inport_15/1 -> SigSpec_15/1
  SigSpec_16/1 -> Outport_16/1
  Inport_16/1 -> SigSpec_16/1
  SigSpec_17/1 -> Outport_17/1
  Inport_17/1 -> SigSpec_17/1
  SigSpec_18/1 -> Outport_18/1
  Inport_18/1 -> SigSpec_18/1
  SigSpec_19/1 -> Outport_19/1
  Inport_19/1 -> SigSpec_19/1
  SigSpec_20/1 -> Outport_20/1
  Inport_20/1 -> SigSpec_20/1
  SigSpec_21/1 -> Outport_21/1
  Inport_21/1 -> SigSpec_21/1
  SigSpec_22/1 -> Outport_22/1
  Inport_22/1 -> SigSpec_22/1
  SigSpec_23/1 -> Outport_23/1
  Inport_23/1 -> SigSpec_23/1
  SigSpec_24/1 -> Outport_24/1
  Inport_24/1 -> SigSpec_24/1
  SigSpec_25/1 -> Outport_25/1
  Inport_25/1 -> SigSpec_25/1
  SigSpec_26/1 -> Outport_26/1
  Inport_26/1 -> SigSpec_26/1
  SigSpec_27/1 -> Outport_27/1
  Inport_27/1 -> SigSpec_27/1
  SigSpec_28/1 -> Outport_28/1
  Inport_28/1 -> SigSpec_28/1

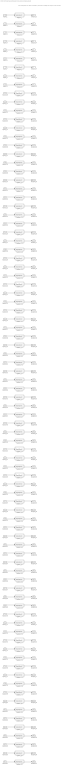
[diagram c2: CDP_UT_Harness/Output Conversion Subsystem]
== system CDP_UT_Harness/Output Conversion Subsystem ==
  note: This subsystem has been inserted by Simulink to adapt the output of the harnessed component to the interface required by the sink blocks. Modifying the contents of this subsystem may result in compilation and simulation failure.
  Inport_1 : Inport
  Inport_2 : Inport  Port=2
  Inport_3 : Inport  Port=3
  Inport_4 : Inport  Port=4
  Inport_5 : Inport  Port=5
  Inport_6 : Inport  Port=6
  Inport_7 : Inport  Port=7
  Inport_8 : Inport  Port=8
  Inport_9 : Inport  Port=9
  Inport_10 : Inport  Port=10
  Inport_11 : Inport  Port=11
  Inport_12 : Inport  Port=12
  Inport_13 : Inport  Port=13
  Inport_14 : Inport  Port=14
  Inport_15 : Inport  Port=15
  Inport_16 : Inport  Port=16
  Inport_17 : Inport  Port=17
  Inport_18 : Inport  Port=18
  Inport_19 : Inport  Port=19
  Inport_20 : Inport  Port=20
  Inport_21 : Inport  Port=21
  Inport_22 : Inport  Port=22
  Inport_23 : Inport  Port=23
  Inport_24 : Inport  Port=24
  Inport_25 : Inport  Port=25
  Inport_26 : Inport  Port=26
  Inport_27 : Inport  Port=27
  Inport_28 : Inport  Port=28
  Inport_29 : Inport  Port=29
  Inport_30 : Inport  Port=30
  Inport_31 : Inport  Port=31
  Inport_32 : Inport  Port=32
  Inport_33 : Inport  Port=33
  Inport_34 : Inport  Port=34
  Inport_35 : Inport  Port=35
  Inport_36 : Inport  Port=36
  Inport_37 : Inport  Port=37
  Inport_38 : Inport  Port=38
  Inport_39 : Inport  Port=39
  Inport_40 : Inport  Port=40
  Inport_41 : Inport  Port=41
  Inport_42 : Inport  Port=42
  Inport_43 : Inport  Port=43
  Inport_44 : Inport  Port=44
  Inport_45 : Inport  Port=45
  Inport_46 : Inport  Port=46
  Inport_47 : Inport  Port=47
  Inport_48 : Inport  Port=48
  Inport_49 : Inport  Port=49
  Inport_50 : Inport  Port=50
  Inport_51 : Inport  Port=51
  Inport_52 : Inport  Port=52
  Inport_53 : Inport  Port=53
  Inport_54 : Inport  Port=54
  Inport_55 : Inport  Port=55
  Inport_56 : Inport  Port=56
  Inport_57 : Inport  Port=57
  Inport_58 : Inport  Port=58
  Inport_59 : Inport  Port=59
  Inport_60 : Inport  Port=60
  Inport_61 : Inport  Port=61
  Inport_62 : Inport  Port=62
  Inport_63 : Inport  Port=63
  Inport_64 : Inport  Port=64
  Inport_65 : Inport  Port=65
  Inport_66 : Inport  Port=66
  Inport_67 : Inport  Port=67
  Inport_68 : Inport  Port=68
  Inport_69 : Inport  Port=69
  Inport_70 : Inport  Port=70
  Inport_71 : Inport  Port=71
  Inport_72 : Inport  Port=72
  Inport_73 : Inport  Port=73
  Inport_74 : Inport  Port=74
  Inport_75 : Inport  Port=75
  Inport_76 : Inport  Port=76
  Inport_77 : Inport  Port=77
  Inport_78 : Inport  Port=78
  Inport_79 : Inport  Port=79
  Inport_80 : Inport  Port=80
  Inport_81 : Inport  Port=81
  Inport_82 : Inport  Port=82
  Inport_83 : Inport  Port=83
  Inport_84 : Inport  Port=84
  Inport_85 : Inport  Port=85
  Inport_86 : Inport  Port=86
  Inport_87 : Inport  Port=87
  SigSpec_1 : SignalSpecification  OutDataTypeStr=single  Unit=V  Dimensions=[1]  SampleTime=0.01
  SigSpec_{7,10,13,21,27,33,37,43..63,71..87} (45 alike) : SignalSpecification  OutDataTypeStr=boolean  Unit=flag  Dimensions=[1]  SampleTime=0.01
  SigSpec_11 : SignalSpecification  OutDataTypeStr=boolean  Unit=flag  Dimensions=[16]  SampleTime=0.01
  SigSpec_12 : SignalSpecification  OutDataTypeStr=boolean  Unit=flag  Dimensions=[16]  SampleTime=0.01
  SigSpec_{14..15,20,23,25,38..39,42,67..68} (10 alike) : SignalSpecification  OutDataTypeStr=single  Unit=C  Dimensions=[1]  SampleTime=0.01
  SigSpec_{2..3,16,18,24,26,40..41,69..70} (10 alike) : SignalSpecification  OutDataTypeStr=uint8  Unit=numb  Dimensions=[1]  SampleTime=0.01
  SigSpec_17 : SignalSpecification  OutDataTypeStr=single  Unit=C  Dimensions=[48]  SampleTime=0.01
  SigSpec_19 : SignalSpecification  OutDataTypeStr=boolean  Unit=flag  Dimensions=[48]  SampleTime=0.01
  SigSpec_22 : SignalSpecification  OutDataTypeStr=boolean  Unit=flag  Dimensions=[16]
  SigSpec_28 : SignalSpecification  OutDataTypeStr=boolean  Unit=flg  Dimensions=[112]  SampleTime=0.01
  SigSpec_29 : SignalSpecification  OutDataTypeStr=boolean  Unit=flg  Dimensions=[112]  SampleTime=0.01
  SigSpec_30 : SignalSpecification  OutDataTypeStr=boolean  Unit=flg  Dimensions=[112]  SampleTime=0.01
  SigSpec_31 : SignalSpecification  OutDataTypeStr=boolean  Unit=flag  Dimensions=[32]  SampleTime=0.01
  SigSpec_32 : SignalSpecification  OutDataTypeStr=single  Unit=C  Dimensions=[32]  SampleTime=0.01
  SigSpec_34 : SignalSpecification  OutDataTypeStr=single  Unit=V  Dimensions=[1]  SampleTime=0.01
  SigSpec_35 : SignalSpecification  OutDataTypeStr=single  Unit=C  Dimensions=[48]  SampleTime=0.01
  SigSpec_36 : SignalSpecification  OutDataTypeStr=boolean  Unit=flag  Dimensions=[48]  SampleTime=0.01
  SigSpec_4 : SignalSpecification  OutDataTypeStr=uint16  Unit=mV  Dimensions=[1]  SampleTime=0.01
  SigSpec_5 : SignalSpecification  OutDataTypeStr=uint16  Unit=mV  Dimensions=[112]  SampleTime=0.01
  SigSpec_6 : SignalSpecification  OutDataTypeStr=boolean  Unit=flag  Dimensions=[112]  SampleTime=0.01
  SigSpec_64 : SignalSpecification  OutDataTypeStr=uint16  Unit=mV  Dimensions=[16]  SampleTime=0.01
  SigSpec_65 : SignalSpecification  OutDataTypeStr=boolean  Unit=flag  Dimensions=[8]  SampleTime=0.01
  SigSpec_66 : SignalSpecification  OutDataTypeStr=single  Unit=C  Dimensions=[8]  SampleTime=0.01
  SigSpec_8 : SignalSpecification  OutDataTypeStr=uint16  Unit=mV  Dimensions=[1]  SampleTime=0.01
  SigSpec_9 : SignalSpecification  OutDataTypeStr=uint16  Unit=mV  Dimensions=[1]  SampleTime=0.01
  Outport_1 : Outport
  Outport_2 : Outport  Port=2
  Outport_3 : Outport  Port=3
  Outport_4 : Outport  Port=4
  Outport_5 : Outport  Port=5
  Outport_6 : Outport  Port=6
  Outport_7 : Outport  Port=7
  Outport_8 : Outport  Port=8
  Outport_9 : Outport  Port=9
  Outport_10 : Outport  Port=10
  Outport_11 : Outport  Port=11
  Outport_12 : Outport  Port=12
  Outport_13 : Outport  Port=13
  Outport_14 : Outport  Port=14
  Outport_15 : Outport  Port=15
  Outport_16 : Outport  Port=16
  Outport_17 : Outport  Port=17
  Outport_18 : Outport  Port=18
  Outport_19 : Outport  Port=19
  Outport_20 : Outport  Port=20
  Outport_21 : Outport  Port=21
  Outport_22 : Outport  Port=22
  Outport_23 : Outport  Port=23
  Outport_24 : Outport  Port=24
  Outport_25 : Outport  Port=25
  Outport_26 : Outport  Port=26
  Outport_27 : Outport  Port=27
  Outport_28 : Outport  Port=28
  Outport_29 : Outport  Port=29
  Outport_30 : Outport  Port=30
  Outport_31 : Outport  Port=31
  Outport_32 : Outport  Port=32
  Outport_33 : Outport  Port=33
  Outport_34 : Outport  Port=34
  Outport_35 : Outport  Port=35
  Outport_36 : Outport  Port=36
  Outport_37 : Outport  Port=37
  Outport_38 : Outport  Port=38
  Outport_39 : Outport  Port=39
  Outport_40 : Outport  Port=40
  Outport_41 : Outport  Port=41
  Outport_42 : Outport  Port=42
  Outport_43 : Outport  Port=43
  Outport_44 : Outport  Port=44
  Outport_45 : Outport  Port=45
  Outport_46 : Outport  Port=46
  Outport_47 : Outport  Port=47
  Outport_48 : Outport  Port=48
  Outport_49 : Outport  Port=49
  Outport_50 : Outport  Port=50
  Outport_51 : Outport  Port=51
  Outport_52 : Outport  Port=52
  Outport_53 : Outport  Port=53
  Outport_54 : Outport  Port=54
  Outport_55 : Outport  Port=55
  Outport_56 : Outport  Port=56
  Outport_57 : Outport  Port=57
  Outport_58 : Outport  Port=58
  Outport_59 : Outport  Port=59
  Outport_60 : Outport  Port=60
  Outport_61 : Outport  Port=61
  Outport_62 : Outport  Port=62
  Outport_63 : Outport  Port=63
  Outport_64 : Outport  Port=64
  Outport_65 : Outport  Port=65
  Outport_66 : Outport  Port=66
  Outport_67 : Outport  Port=67
  Outport_68 : Outport  Port=68
  Outport_69 : Outport  Port=69
  Outport_70 : Outport  Port=70
  Outport_71 : Outport  Port=71
  Outport_72 : Outport  Port=72
  Outport_73 : Outport  Port=73
  Outport_74 : Outport  Port=74
  Outport_75 : Outport  Port=75
  Outport_76 : Outport  Port=76
  Outport_77 : Outport  Port=77
  Outport_78 : Outport  Port=78
  Outport_79 : Outport  Port=79
  Outport_80 : Outport  Port=80
  Outport_81 : Outport  Port=81
  Outport_82 : Outport  Port=82
  Outport_83 : Outport  Port=83
  Outport_84 : Outport  Port=84
  Outport_85 : Outport  Port=85
  Outport_86 : Outport  Port=86
  Outport_87 : Outport  Port=87
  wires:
  Inport_1/1 -> SigSpec_1/1
  SigSpec_1/1 -> Outport_1/1
  Inport_2/1 -> SigSpec_2/1
  SigSpec_2/1 -> Outport_2/1
  Inport_3/1 -> SigSpec_3/1
  SigSpec_3/1 -> Outport_3/1
  Inport_4/1 -> SigSpec_4/1
  SigSpec_4/1 -> Outport_4/1
  Inport_5/1 -> SigSpec_5/1
  SigSpec_5/1 -> Outport_5/1
  Inport_6/1 -> SigSpec_6/1
  SigSpec_6/1 -> Outport_6/1
  Inport_7/1 -> SigSpec_7/1
  SigSpec_7/1 -> Outport_7/1
  Inport_8/1 -> SigSpec_8/1
  SigSpec_8/1 -> Outport_8/1
  Inport_9/1 -> SigSpec_9/1
  SigSpec_9/1 -> Outport_9/1
  Inport_10/1 -> SigSpec_10/1
  SigSpec_10/1 -> Outport_10/1
  Inport_11/1 -> SigSpec_11/1
  SigSpec_11/1 -> Outport_11/1
  Inport_12/1 -> SigSpec_12/1
  SigSpec_12/1 -> Outport_12/1
  Inport_13/1 -> SigSpec_13/1
  SigSpec_13/1 -> Outport_13/1
  Inport_14/1 -> SigSpec_14/1
  SigSpec_14/1 -> Outport_14/1
  Inport_15/1 -> SigSpec_15/1
  SigSpec_15/1 -> Outport_15/1
  Inport_16/1 -> SigSpec_16/1
  SigSpec_16/1 -> Outport_16/1
  Inport_17/1 -> SigSpec_17/1
  SigSpec_17/1 -> Outport_17/1
  Inport_18/1 -> SigSpec_18/1
  SigSpec_18/1 -> Outport_18/1
  Inport_19/1 -> SigSpec_19/1
  SigSpec_19/1 -> Outport_19/1
  Inport_20/1 -> SigSpec_20/1
  SigSpec_20/1 -> Outport_20/1
  Inport_21/1 -> SigSpec_21/1
  SigSpec_21/1 -> Outport_21/1
  Inport_22/1 -> SigSpec_22/1
  SigSpec_22/1 -> Outport_22/1
  Inport_23/1 -> SigSpec_23/1
  SigSpec_23/1 -> Outport_23/1
  Inport_24/1 -> SigSpec_24/1
  SigSpec_24/1 -> Outport_24/1
  Inport_25/1 -> SigSpec_25/1
  SigSpec_25/1 -> Outport_25/1
  Inport_26/1 -> SigSpec_26/1
  SigSpec_26/1 -> Outport_26/1
  Inport_27/1 -> SigSpec_27/1
  SigSpec_27/1 -> Outport_27/1
  Inport_28/1 -> SigSpec_28/1
  SigSpec_28/1 -> Outport_28/1
  Inport_29/1 -> SigSpec_29/1
  SigSpec_29/1 -> Outport_29/1
  Inport_30/1 -> SigSpec_30/1
  SigSpec_30/1 -> Outport_30/1
  Inport_31/1 -> SigSpec_31/1
  SigSpec_31/1 -> Outport_31/1
  Inport_32/1 -> SigSpec_32/1
  SigSpec_32/1 -> Outport_32/1
  Inport_33/1 -> SigSpec_33/1
  SigSpec_33/1 -> Outport_33/1
  Inport_34/1 -> SigSpec_34/1
  SigSpec_34/1 -> Outport_34/1
  Inport_35/1 -> SigSpec_35/1
  SigSpec_35/1 -> Outport_35/1
  Inport_36/1 -> SigSpec_36/1
  SigSpec_36/1 -> Outport_36/1
  Inport_37/1 -> SigSpec_37/1
  SigSpec_37/1 -> Outport_37/1
  Inport_38/1 -> SigSpec_38/1
  SigSpec_38/1 -> Outport_38/1
  Inport_39/1 -> SigSpec_39/1
  SigSpec_39/1 -> Outport_39/1
  Inport_40/1 -> SigSpec_40/1
  SigSpec_40/1 -> Outport_40/1
  Inport_41/1 -> SigSpec_41/1
  SigSpec_41/1 -> Outport_41/1
  Inport_42/1 -> SigSpec_42/1
  SigSpec_42/1 -> Outport_42/1
  Inport_43/1 -> SigSpec_43/1
  SigSpec_43/1 -> Outport_43/1
  Inport_44/1 -> SigSpec_44/1
  SigSpec_44/1 -> Outport_44/1
  Inport_45/1 -> SigSpec_45/1
  SigSpec_45/1 -> Outport_45/1
  Inport_46/1 -> SigSpec_46/1
  SigSpec_46/1 -> Outport_46/1
  Inport_47/1 -> SigSpec_47/1
  SigSpec_47/1 -> Outport_47/1
  Inport_48/1 -> SigSpec_48/1
  SigSpec_48/1 -> Outport_48/1
  Inport_49/1 -> SigSpec_49/1
  SigSpec_49/1 -> Outport_49/1
  Inport_50/1 -> SigSpec_50/1
  SigSpec_50/1 -> Outport_50/1
  Inport_51/1 -> SigSpec_51/1
  SigSpec_51/1 -> Outport_51/1
  Inport_52/1 -> SigSpec_52/1
  SigSpec_52/1 -> Outport_52/1
  Inport_53/1 -> SigSpec_53/1
  SigSpec_53/1 -> Outport_53/1
  Inport_54/1 -> SigSpec_54/1
  SigSpec_54/1 -> Outport_54/1
  Inport_55/1 -> SigSpec_55/1
  SigSpec_55/1 -> Outport_55/1
  Inport_56/1 -> SigSpec_56/1
  SigSpec_56/1 -> Outport_56/1
  Inport_57/1 -> SigSpec_57/1
  SigSpec_57/1 -> Outport_57/1
  Inport_58/1 -> SigSpec_58/1
  SigSpec_58/1 -> Outport_58/1
  Inport_59/1 -> SigSpec_59/1
  SigSpec_59/1 -> Outport_59/1
  Inport_60/1 -> SigSpec_60/1
  SigSpec_60/1 -> Outport_60/1
  Inport_61/1 -> SigSpec_61/1
  SigSpec_61/1 -> Outport_61/1
  Inport_62/1 -> SigSpec_62/1
  SigSpec_62/1 -> Outport_62/1
  Inport_63/1 -> SigSpec_63/1
  SigSpec_63/1 -> Outport_63/1
  Inport_64/1 -> SigSpec_64/1
  SigSpec_64/1 -> Outport_64/1
  Inport_65/1 -> SigSpec_65/1
  SigSpec_65/1 -> Outport_65/1
  Inport_66/1 -> SigSpec_66/1
  SigSpec_66/1 -> Outport_66/1
  Inport_67/1 -> SigSpec_67/1
  SigSpec_67/1 -> Outport_67/1
  Inport_68/1 -> SigSpec_68/1
  SigSpec_68/1 -> Outport_68/1
  Inport_69/1 -> SigSpec_69/1
  SigSpec_69/1 -> Outport_69/1
  Inport_70/1 -> SigSpec_70/1
  SigSpec_70/1 -> Outport_70/1
  Inport_71/1 -> SigSpec_71/1
  SigSpec_71/1 -> Outport_71/1
  Inport_72/1 -> SigSpec_72/1
  SigSpec_72/1 -> Outport_72/1
  Inport_73/1 -> SigSpec_73/1
  SigSpec_73/1 -> Outport_73/1
  Inport_74/1 -> SigSpec_74/1
  SigSpec_74/1 -> Outport_74/1
  Inport_75/1 -> SigSpec_75/1
  SigSpec_75/1 -> Outport_75/1
  Inport_76/1 -> SigSpec_76/1
  SigSpec_76/1 -> Outport_76/1
  Inport_77/1 -> SigSpec_77/1
  SigSpec_77/1 -> Outport_77/1
  Inport_78/1 -> SigSpec_78/1
  SigSpec_78/1 -> Outport_78/1
  Inport_79/1 -> SigSpec_79/1
  SigSpec_79/1 -> Outport_79/1
  Inport_80/1 -> SigSpec_80/1
  SigSpec_80/1 -> Outport_80/1
  Inport_81/1 -> SigSpec_81/1
  SigSpec_81/1 -> Outport_81/1
  Inport_82/1 -> SigSpec_82/1
  SigSpec_82/1 -> Outport_82/1
  Inport_83/1 -> SigSpec_83/1
  SigSpec_83/1 -> Outport_83/1
  Inport_84/1 -> SigSpec_84/1
  SigSpec_84/1 -> Outport_84/1
  Inport_85/1 -> SigSpec_85/1
  SigSpec_85/1 -> Outport_85/1
  Inport_86/1 -> SigSpec_86/1
  SigSpec_86/1 -> Outport_86/1
  Inport_87/1 -> SigSpec_87/1
  SigSpec_87/1 -> Outport_87/1
